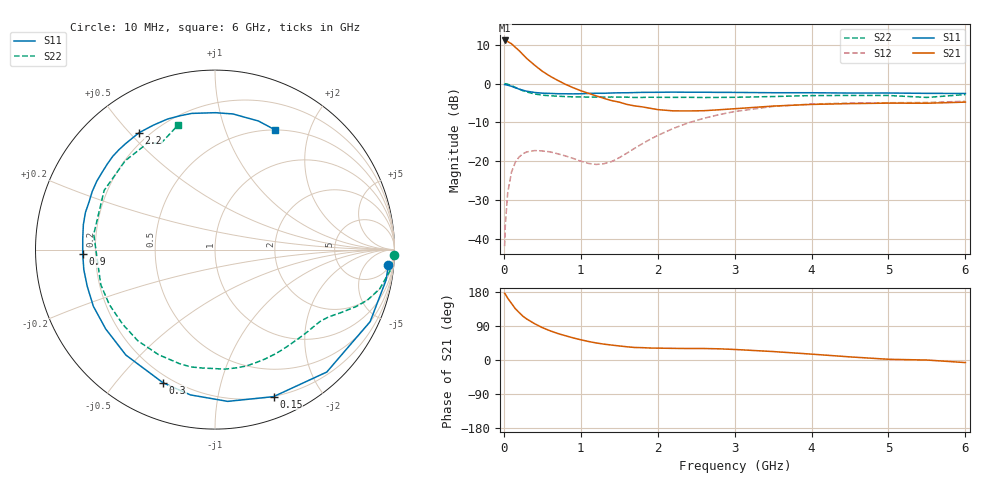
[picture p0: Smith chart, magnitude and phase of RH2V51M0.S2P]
! SIEMENS Small Signal Semiconductors
! BFR106
! Si NPN RF Bipolar Junction Transistor in SOT23
! VCE = 2.5 V  IC = 1 mA
! Common Emitter S-Parameters:  August  1996
# GHz  S  MA  R  50
!  f  S11  S21  S12  S22
! GHz  MAG  ANG  MAG  ANG  MAG  ANG  MAG  ANG
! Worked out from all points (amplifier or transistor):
!   36 points, 10 MHz to 6 GHz, reference 50 ohm
!   highest |S21| = 11.1 dB at 10 MHz (marker M1)
!   |S21| within 3 dB of that: start of sweep to 217.1 MHz
!   unconditionally stable (mu >= 1): 857.6 MHz to end of sweep
!   at 250 MHz: K = 0.27, MSG = 12.8 dB, |S12| = -18.1 dB
!   at 1.4 GHz: K = 1.50, MAG = 3.7 dB, |S12| = -20.1 dB
!   at 6 GHz: K = 1.02, MAG = -1.0 dB, |S12| = -4.6 dB
!   S11 on the Smith chart (normalised r, x): 10 MHz: 7, -20; 150 MHz: 0.20, -1.46; 300 MHz: 0.17, -0.67; 900 MHz: 0.15, -0.02; 2.2 GHz: 0.16, +0.53; 6 GHz: 0.50, +1.51
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0.01  0.9698 -5.1  3.602 176.0  0.008 88.9  0.9993 -1.6
0.02  0.9682 -10.1  3.578 173.5  0.0153 84.1  0.9959 -2.9
0.05  0.953 -24.9  3.484 163.2  0.0389 75.8  0.9808 -7.1
0.1  0.9237 -47.6  3.263 149.2  0.0724 63.5  0.9432 -13.4
0.15  0.8817 -68.3  2.937 135.2  0.0972 51.6  0.8942 -18.4
0.2  0.8486 -85.2  2.655 125.0  0.1136 43.4  0.8491 -21.9
0.25  0.8211 -99.6  2.359 115.2  0.1249 36.2  0.8075 -24.8
0.3  0.7966 -111.3  2.101 107.9  0.1316 31.1  0.7792 -27.0
0.4  0.7692 -130.2  1.729 95.8  0.1368 22.9  0.735 -30.7
0.5  0.7525 -144.0  1.444 85.5  0.1354 17.7  0.7095 -34.3
0.7  0.7407 -164.0  1.101 70.0  0.1244 12.8  0.6878 -42.4
0.9  0.7374 -178.2  0.886 58.4  0.1085 14.7  0.6747 -50.8
1.1  0.7465 169.3  0.75 48.9  0.0934 24.8  0.6711 -60.2
1.3  0.7503 159.1  0.646 41.9  0.0926 42.8  0.6696 -70.0
1.6  0.762 145.9  0.539 34.9  0.1268 64.6  0.6684 -85.3
2.2  0.7766 123.1  0.445 30.7  0.2635 67.3  0.6646 -118.3
2.8  0.7708 104.7  0.46 29.5  0.3982 52.9  0.6636 -152.5
3.5  0.7628 89.9  0.513 22.3  0.5075 34.7  0.6809 172.8
4.5  0.7554 76.6  0.552 8.2  0.5609 13.3  0.7038 135.3
5  0.7563 71.4  0.56 1.9  0.5663 5.6  0.7027 121.9
5.5  0.7485 66.5  0.558 -0.1  0.5708 2.0  0.6633 117.2
6  0.7459 63.2  0.577 -6.8  0.592 -5.6  0.7222 106.7
